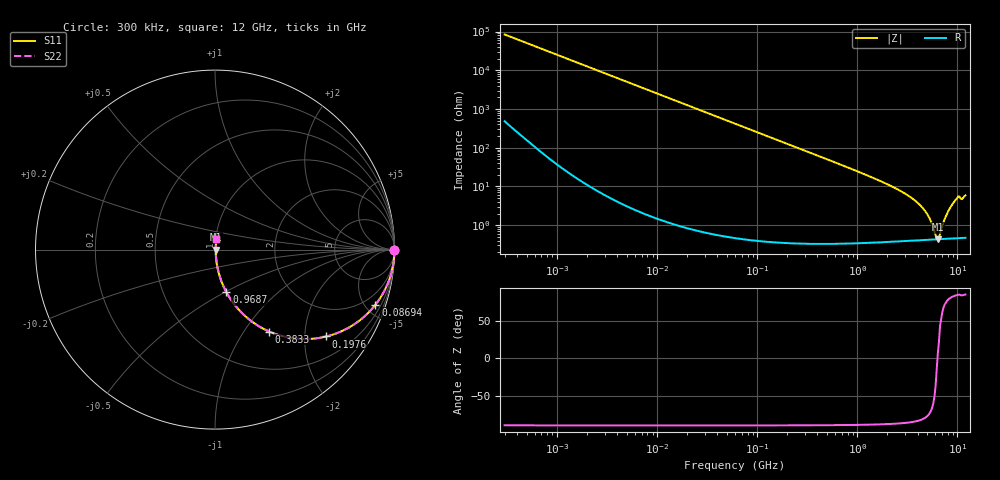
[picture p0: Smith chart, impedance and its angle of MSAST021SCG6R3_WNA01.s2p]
! MSAST021SCG6R3_WNA01  S-PARAMETER MODEL  ( General Type )
! Model Generated by TAIYO YUDEN Corporation (http://www.ty-top.com)
! Version 2.0
! TAIYO YUDEN Control No. 181101
! Copyright(c) 2015 TAIYO YUDEN CO.,LTD. All Rights Reserved.
! Product Description (link to TY-COMPAS)
! https://ds.yuden.co.jp/TYCOMPAS/or/detail?pn=MSAST021SCG6R3CWNA01&u=M
! Products Name : Multilayer Ceramic Capacitors
! Characteristics :
!  Capacitance : 6.3 pF , Rated Voltage : 25V , TCC : CG / C0G
!  Case Size : 0.25 x 0.125 / 0.0098 x 0.0049 [mm/inch] , Thickness : 0.125 / 0.0049 [mm/inch]
!  (Conditions: Temperature = 25 degC , DC Bias Current/Voltage = 0A / 0V)
! External Node Assignments :
!  1  o---| |---o  2
! GND o---------o GND
! Frequency Range : 0.3MHz  -  12000MHz  [ 401 STEP ]
# MHz S RI R 50
! Freq[MHz].  S11 Real  S11 Imag  S21 Real  S21 Imag  S12 Real  S12 Imag  S22 Real  S22 Imag
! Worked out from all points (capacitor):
!   401 points, 300 kHz to 12 GHz, reference 50 ohm
!   read as one part in series: C = 6.3 pF near 316.3 kHz
!   lowest |Z| = 436 mohm at 6.354 GHz (marker M1)
!   series resonance near 6.319 GHz, so ESL is about 100 pH
!   S11 on the Smith chart (normalised r, x): 300 kHz: open; 86.94 MHz: 1.01, -5.81; 197.6 MHz: 1.01, -2.55; 383.3 MHz: 1.01, -1.31; 968.7 MHz: 1.01, -0.51; 12 GHz: 1.01, +0.12
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0.3  1 -0.00119  8.21e-06 0.00119  8.21e-06 0.00119  1 -0.00119
1.769972  0.9999 -0.00701  5.56e-05 0.00701  5.56e-05 0.00701  0.9999 -0.00701
10.44266  0.9983 -0.0413  0.00173 0.0413  0.00173 0.0413  0.9983 -0.0413
27.82928  0.9879 -0.1088  0.0121 0.1088  0.0121 0.1088  0.9879 -0.1088
60  0.9464 -0.2247  0.0536 0.2247  0.0536 0.2247  0.9464 -0.2247
86.94074  0.8937 -0.3075  0.1063 0.3075  0.1063 0.3075  0.8937 -0.3075
197.6437  0.6195 -0.4842  0.3805 0.4842  0.3805 0.4842  0.6195 -0.4842
353.9943  0.3367 -0.4703  0.6633 0.4703  0.6633 0.4703  0.3367 -0.4703
383.2761  0.3022 -0.4567  0.6978 0.4567  0.6978 0.4567  0.3022 -0.4567
601.3112  0.1497 -0.3528  0.8503 0.3528  0.8503 0.3528  0.1497 -0.3528
968.706  0.0637 -0.2376  0.9363 0.2376  0.9363 0.2376  0.0637 -0.2376
2088.533  0.015 -0.1056  0.985 0.1056  0.985 0.1056  0.015 -0.1056
3190.978  0.00732 -0.0582  0.9927 0.0582  0.9927 0.0582  0.00732 -0.0582
4270.516  0.00509 -0.0317  0.9949 0.0317  0.9949 0.0317  0.00509 -0.0317
5140.631  0.00446 -0.0163  0.9955 0.0163  0.9955 0.0163  0.00446 -0.0163
6026.253  0.0043 -0.00351  0.9957 0.00351  0.9957 0.00351  0.0043 -0.00351
6354.153  0.00432 0.000377  0.9957 -0.000377  0.9957 -0.000377  0.00432 0.000377
6699.894  0.00437 0.00412  0.9956 -0.00412  0.9956 -0.00412  0.00437 0.00412
7854.144  0.00481 0.0189  0.9952 -0.0189  0.9952 -0.0189  0.00481 0.0189
8966.534  0.00575 0.0349  0.9942 -0.0349  0.9942 -0.0349  0.00575 0.0349
9968.853  0.00709 0.0498  0.9929 -0.0498  0.9929 -0.0498  0.00709 0.0498
12000  0.00809 0.0579  0.9919 -0.0579  0.9919 -0.0579  0.00809 0.0579
